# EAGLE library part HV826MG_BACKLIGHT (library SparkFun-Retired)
Small EL backlight driver for the CFAX 128x64 graphical display.
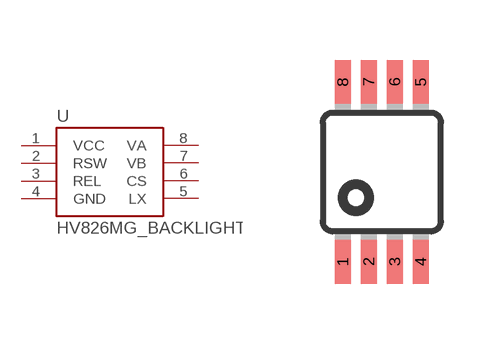
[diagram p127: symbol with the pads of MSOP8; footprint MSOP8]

Designator prefix -

## HV826MG_BACKLIGHT  [MSOP8]
1  VCC
2  RSW
3  REL  pwr
4  GND  pwr
5  LX
6  CS
7  VB
8  VA

## Footprint MSOP8 (pad centres in mm)
8M, 8-Lead, 0.118" Wide, Miniature Small Outline Package MSOP 8M-Package doc1097.pdf
smd 0.4 x 1.1: 1 -0.975,-2.25; 2 -0.325,-2.25; 3 0.325,-2.25; 4 0.975,-2.25; 5 0.975,2.25; 6 0.325,2.25; 7 -0.325,2.25; 8 -0.975,2.25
